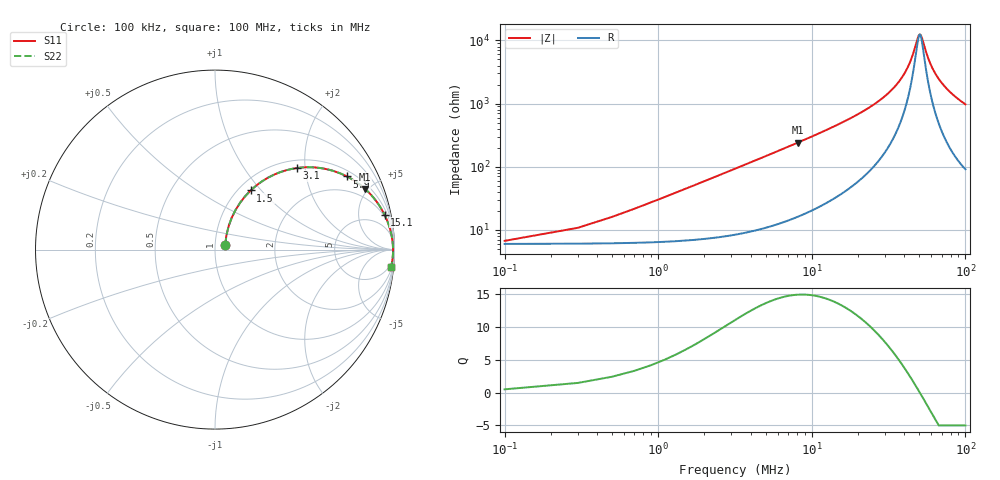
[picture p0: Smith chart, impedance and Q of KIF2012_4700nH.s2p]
!version-2
!date-12.2020
!Series
# MHz S RI R 50
!Freq ReS11 ImS11 ReS21 ImS21 ReS12 ImS12 ReS22 ImS22
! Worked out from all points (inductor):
!   501 points, 100 kHz to 100 MHz, reference 50 ohm
!   read as one part in series: L = 4.67 uH near 700 kHz
!   highest Q = 14.9 at 8.1 MHz (marker M1), where L = 4.7 uH
!   self-resonance near 50.51 MHz
!   S11 on the Smith chart (normalised r, x): 100 kHz: 1.12, +0.06; 1.5 MHz: 1.13, +0.88; 3.1 MHz: 1.17, +1.81; 5.9 MHz: 1.24, +3.45; 15.1 MHz: 1.70, +9.48; 100 MHz: 3, -19
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0.1  0.057 0.0266  0.943 -0.0266  0.943 -0.0266  0.057 0.0266
0.9  0.1142 0.2203  0.8858 -0.2203  0.8858 -0.2203  0.1142 0.2203
1.5  0.1987 0.3296  0.8013 -0.3296  0.8013 -0.3296  0.1987 0.3296
2.3  0.3306 0.4183  0.6694 -0.4183  0.6694 -0.4183  0.3306 0.4183
3.1  0.4557 0.4544  0.5443 -0.4544  0.5443 -0.4544  0.4557 0.4544
4.5  0.6251 0.4474  0.3749 -0.4474  0.3749 -0.4474  0.6251 0.4474
5.9  0.7356 0.4074  0.2644 -0.4074  0.2644 -0.4074  0.7356 0.4074
8.1  0.836 0.3383  0.164 -0.3383  0.164 -0.3383  0.836 0.3383
15.1  0.9444 0.1951  0.0556 -0.1951  0.0556 -0.1951  0.9444 0.1951
16.9  0.9549 0.1722  0.0451 -0.1722  0.0451 -0.1722  0.9549 0.1722
33.5  0.9875 0.0572  0.0125 -0.0572  0.0125 -0.0572  0.9875 0.0572
42.1  0.991 0.025  0.00901 -0.025  0.00901 -0.025  0.991 0.025
45.1  0.9916 0.0155  0.00845 -0.0155  0.00845 -0.0155  0.9916 0.0155
48.9  0.9919 0.00442  0.00806 -0.00442  0.00806 -0.00442  0.9919 0.00442
50.1  0.992 0.00111  0.008 -0.00111  0.008 -0.00111  0.992 0.00111
51.7  0.992 -0.00319  0.00797 0.00319  0.00797 0.00319  0.992 -0.00319
55.9  0.9919 -0.0139  0.00808 0.0139  0.00808 0.0139  0.9919 -0.0139
59.1  0.9917 -0.0216  0.00834 0.0216  0.00834 0.0216  0.9917 -0.0216
66.7  0.9906 -0.0385  0.00942 0.0385  0.00942 0.0385  0.9906 -0.0385
74.1  0.989 -0.0535  0.011 0.0535  0.011 0.0535  0.989 -0.0535
83.5  0.9863 -0.0713  0.0137 0.0713  0.0137 0.0713  0.9863 -0.0713
100  0.9804 -0.0996  0.0196 0.0996  0.0196 0.0996  0.9804 -0.0996
